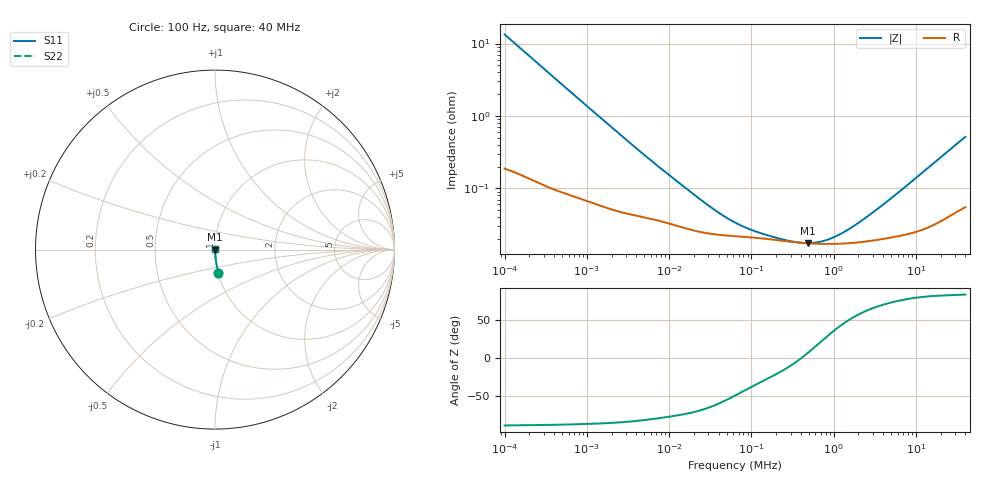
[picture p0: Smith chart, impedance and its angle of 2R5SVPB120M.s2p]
! *  *** Spice model ***
! *  Copyright (C) Panasonic Industry
! *  Conductive Polymer Aluminum Solid Capacitors (OS-CON)
! *  Parts No. 2R5SVPB120M
! Touchstone file from project
# GHZ S RI R 50.000000
! Modal data exported
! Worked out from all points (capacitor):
!   450 points, 100 Hz to 40 MHz, reference 50 ohm
!   read as one part in series: C = 119 uF near 105.9 Hz
!   lowest |Z| = 17.5 mohm at 487 kHz (marker M1)
!   series resonance near 406.8 kHz, so ESL is about 1.3 nH
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1e-07  0.0192 -0.1305  0.9808 0.1305  0.9808 0.1305  0.0192 -0.1305
1.059254e-07  0.0173 -0.1235  0.9827 0.1235  0.9827 0.1235  0.0173 -0.1235
1.584893e-07  0.00857 -0.0836  0.9914 0.0836  0.9914 0.0836  0.00857 -0.0836
2.511886e-07  0.00404 -0.0532  0.996 0.0532  0.996 0.0532  0.00404 -0.0532
8.659643e-07  0.000957 -0.0157  0.999 0.0157  0.999 0.0157  0.000957 -0.0157
3.447466e-06  0.000451 -0.00408  0.9995 0.00408  0.9995 0.00408  0.000451 -0.00408
7.498942e-06  0.00036 -0.00195  0.9996 0.00195  0.9996 0.00195  0.00036 -0.00195
3.072557e-05  0.000237 -0.000516  0.9998 0.000516  0.9998 0.000516  0.000237 -0.000516
4.59727e-05  0.000225 -0.00035  0.9998 0.00035  0.9998 0.00035  0.000225 -0.00035
6.493816e-05  0.000217 -0.00025  0.9998 0.00025  0.9998 0.00025  0.000217 -0.00025
0.0001029201  0.000209 -0.00016  0.9998 0.00016  0.9998 0.00016  0.000209 -0.00016
0.0001883649  0.000195 -8.24e-05  0.9998 8.24e-05  0.9998 8.24e-05  0.000195 -8.24e-05
0.0003254618  0.000181 -2.44e-05  0.9998 2.44e-05  0.9998 2.44e-05  0.000181 -2.44e-05
0.0004869675  0.000174 2.08e-05  0.9998 -2.08e-05  0.9998 -2.08e-05  0.000174 2.08e-05
0.0005463865  0.000173 3.48e-05  0.9998 -3.48e-05  0.9998 -3.48e-05  0.000173 3.48e-05
0.0006683439  0.000171 6.09e-05  0.9998 -6.09e-05  0.9998 -6.09e-05  0.000171 6.09e-05
0.0008413951  0.000171 9.43e-05  0.9998 -9.43e-05  0.9998 -9.43e-05  0.000171 9.43e-05
0.001029201  0.000171 0.000128  0.9998 -0.000128  0.9998 -0.000128  0.000171 0.000128
0.001295687  0.000172 0.000172  0.9998 -0.000172  0.9998 -0.000172  0.000172 0.000172
0.002238721  0.000182 0.000315  0.9998 -0.000315  0.9998 -0.000315  0.000182 0.000315
0.004731513  0.000207 0.000661  0.9998 -0.000661  0.9998 -0.000661  0.000207 0.000661
0.04  0.000575 0.0051  0.9994 -0.0051  0.9994 -0.0051  0.000575 0.0051
